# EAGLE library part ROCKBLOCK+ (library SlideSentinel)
ROCKBLOCK+ Satcom modem attached to hub used for making web requests can receive emessages for remote configuration commands
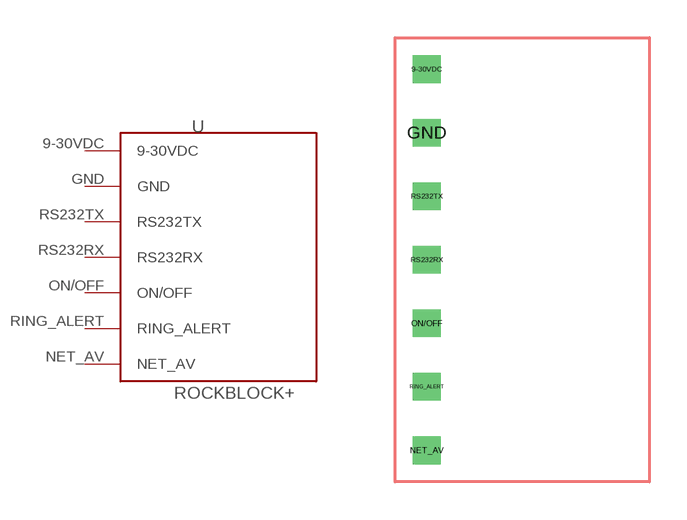
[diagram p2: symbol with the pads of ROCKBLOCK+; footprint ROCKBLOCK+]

Designator prefix -

## ROCKBLOCK+  [ROCKBLOCK+]
9-30VDC  9-30VDC
GND  GND
NET_AV  NET_AV
ON/OFF  ON/OFF
RING_ALERT  RING_ALERT
RS232RX  RS232RX
RS232TX  RS232TX

## Footprint ROCKBLOCK+ (pad centres in mm)
drill 0.6 square: 9-30VDC -13.97,6.35; GND -13.97,3.81; NET_AV -13.97,-8.89; ON/OFF -13.97,-3.81; RING_ALERT -13.97,-6.35; RS232RX -13.97,-1.27; RS232TX -13.97,1.27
